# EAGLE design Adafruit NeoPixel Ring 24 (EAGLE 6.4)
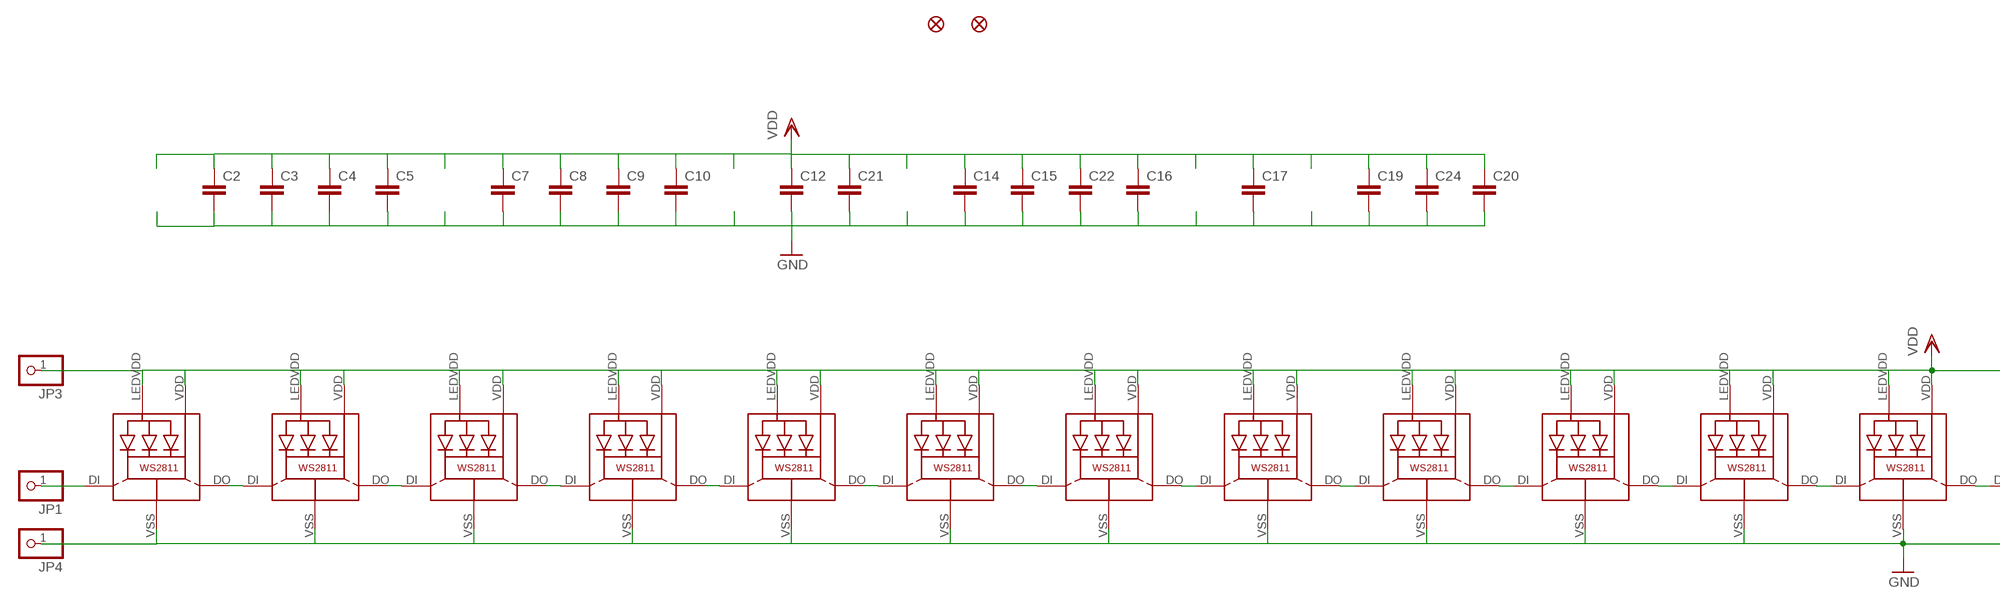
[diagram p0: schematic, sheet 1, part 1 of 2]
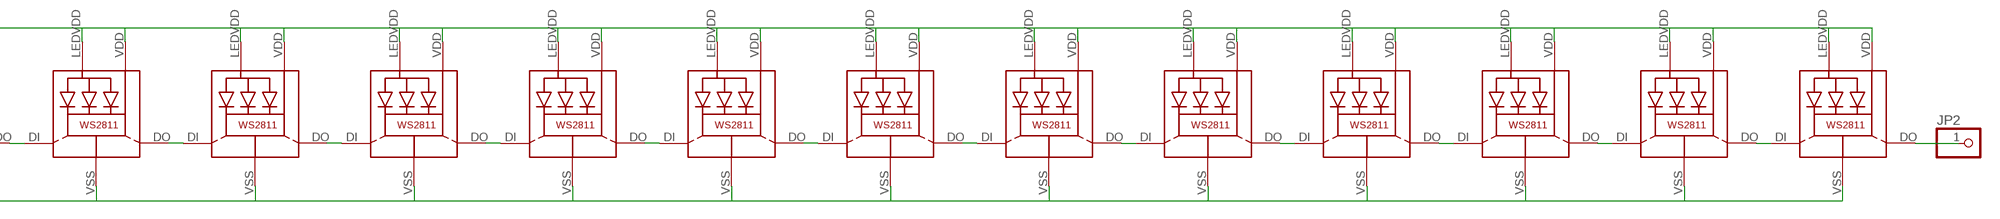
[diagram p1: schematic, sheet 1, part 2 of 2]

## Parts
C2  C-EUC0603  [C0603]
C3  C-EUC0603  [C0603]
C4  C-EUC0603  [C0603]
C5  C-EUC0603  [C0603]
C7  C-EUC0603  [C0603]
C8  C-EUC0603  [C0603]
C9  C-EUC0603  [C0603]
C10  C-EUC0603  [C0603]
C12  C-EUC0603  [C0603]
C14  C-EUC0603  [C0603]
C15  C-EUC0603  [C0603]
C16  C-EUC0603  [C0603]
C17  C-EUC0603  [C0603]
C19  C-EUC0603  [C0603]
C20  C-EUC0603  [C0603]
C21  C-EUC0603  [C0603]
C22  C-EUC0603  [C0603]
C24  C-EUC0603  [C0603]
FID1  FIDUCIAL""  [FIDUCIAL_1MM]
FID2  FIDUCIAL""  [FIDUCIAL_1MM]
JP1  PINHD-1X1CB  [1X01-CLEANBIG]
JP2  PINHD-1X1CB  [1X01-CLEANBIG]
JP3  PINHD-1X1CB  [1X01-CLEANBIG]
JP4  PINHD-1X1CB  [1X01-CLEANBIG]
LED1  WS28115050  [WS28115050]
LED2  WS28115050  [WS28115050]
LED3  WS28115050  [WS28115050]
LED4  WS28115050  [WS28115050]
LED5  WS28115050  [WS28115050]
LED6  WS28115050  [WS28115050]
LED7  WS28115050  [WS28115050]
LED8  WS28115050  [WS28115050]
LED9  WS28115050  [WS28115050]
LED10  WS28115050  [WS28115050]
LED11  WS28115050  [WS28115050]
LED12  WS28115050  [WS28115050]
LED13  WS28115050  [WS28115050]
LED14  WS28115050  [WS28115050]
LED15  WS28115050  [WS28115050]
LED16  WS28115050  [WS28115050]
LED17  WS28115050  [WS28115050]
LED18  WS28115050  [WS28115050]
LED19  WS28115050  [WS28115050]
LED20  WS28115050  [WS28115050]
LED21  WS28115050  [WS28115050]
LED22  WS28115050  [WS28115050]
LED23  WS28115050  [WS28115050]
LED24  WS28115050  [WS28115050]

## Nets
GND: C2.2 C3.2 C4.2 C5.2 C7.2 C8.2 C9.2 C10.2 C12.2 C14.2 C15.2 C16.2 C17.2 C19.2 C20.2 C21.2 C22.2 C24.2 JP4.1 LED1.VSS(GND) LED2.VSS(GND) LED3.VSS(GND) LED4.VSS(GND) LED5.VSS(GND) LED6.VSS(GND) LED7.VSS(GND) LED8.VSS(GND) LED9.VSS(GND) LED10.VSS(GND) LED11.VSS(GND) LED12.VSS(GND) LED13.VSS(GND) LED14.VSS(GND) LED15.VSS(GND) LED16.VSS(GND) LED17.VSS(GND) LED18.VSS(GND) LED19.VSS(GND) LED20.VSS(GND) LED21.VSS(GND) LED22.VSS(GND) LED23.VSS(GND) LED24.VSS(GND)
N$1: LED1.DO LED2.DI
N$2: LED2.DO LED3.DI
N$3: LED3.DO LED4.DI
N$4: LED4.DO LED5.DI
N$5: LED5.DO LED6.DI
N$6: LED6.DO LED7.DI
N$7: LED7.DO LED8.DI
N$8: LED8.DO LED9.DI
N$9: LED9.DO LED10.DI
N$10: LED10.DO LED11.DI
N$11: LED11.DO LED12.DI
N$12: LED12.DO LED13.DI
N$13: LED13.DO LED14.DI
N$14: LED14.DO LED15.DI
N$15: LED15.DO LED16.DI
N$16: LED16.DO LED17.DI
N$17: LED17.DO LED18.DI
N$18: LED18.DO LED19.DI
N$19: LED19.DO LED20.DI
N$20: LED20.DO LED21.DI
N$21: LED21.DO LED22.DI
N$22: LED22.DO LED23.DI
N$23: LED23.DO LED24.DI
N$24: JP2.1 LED24.DO
N$26: JP1.1 LED1.DI
VDD: C2.1 C3.1 C4.1 C5.1 C7.1 C8.1 C9.1 C10.1 C12.1 C14.1 C15.1 C16.1 C17.1 C19.1 C20.1 C21.1 C22.1 C24.1 JP3.1 LED1.LEDVDD LED1.VDD LED2.LEDVDD LED2.VDD LED3.LEDVDD LED3.VDD LED4.LEDVDD LED4.VDD LED5.LEDVDD LED5.VDD LED6.LEDVDD LED6.VDD LED7.LEDVDD LED7.VDD LED8.LEDVDD LED8.VDD LED9.LEDVDD LED9.VDD LED10.LEDVDD LED10.VDD LED11.LEDVDD LED11.VDD LED12.LEDVDD LED12.VDD LED13.LEDVDD LED13.VDD LED14.LEDVDD LED14.VDD LED15.LEDVDD LED15.VDD LED16.LEDVDD LED16.VDD LED17.LEDVDD LED17.VDD LED18.LEDVDD LED18.VDD LED19.LEDVDD LED19.VDD LED20.LEDVDD LED20.VDD LED21.LEDVDD LED21.VDD LED22.LEDVDD LED22.VDD LED23.LEDVDD LED23.VDD LED24.LEDVDD LED24.VDD

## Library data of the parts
C2-C5 C7-C10 C12 C14-C17 C19-C22 C24 = rcl:C-EU: CAPACITOR, European symbol
FID1 FID2 = microbuilder:FIDUCIAL: Fiducial Alignment Points; BOM: EXCLUDE
JP1-JP4 = NeoPixelRing:PINHD-1X1: Pin header 1x1 for 0.1" spacing
LED1-LED24 = microbuilder:WS28115050

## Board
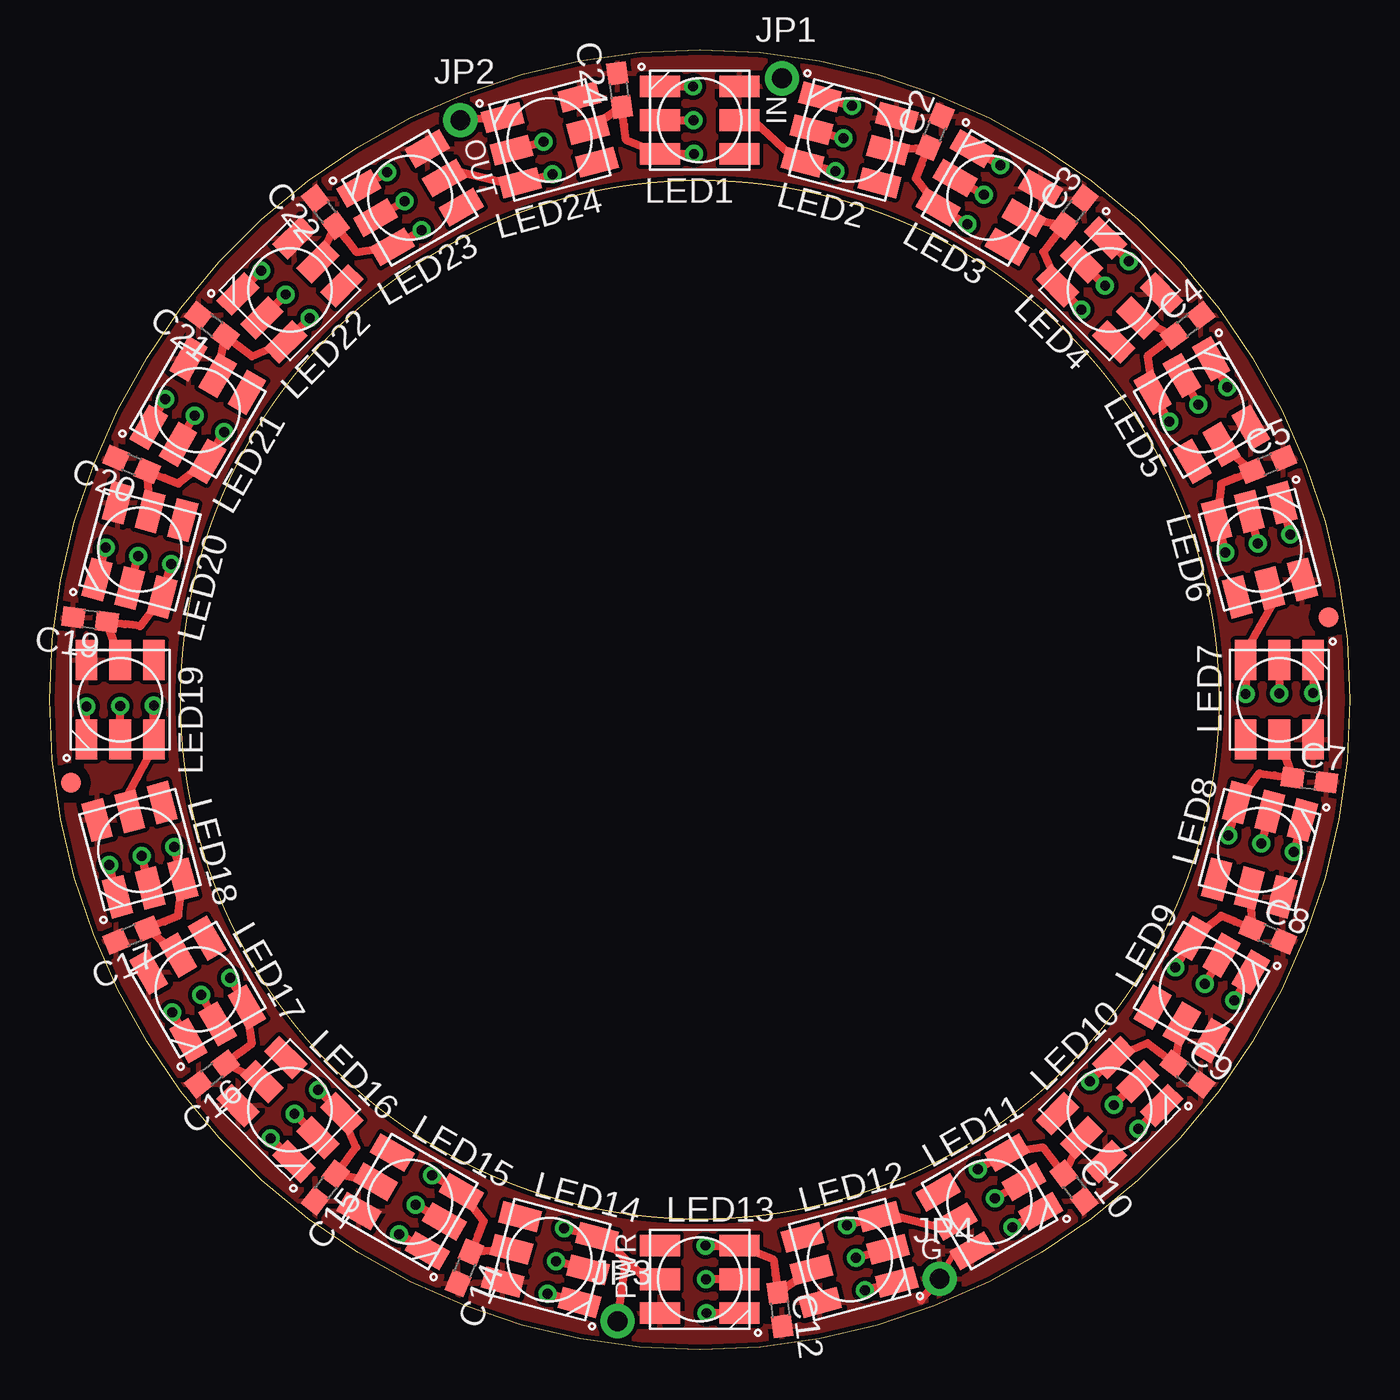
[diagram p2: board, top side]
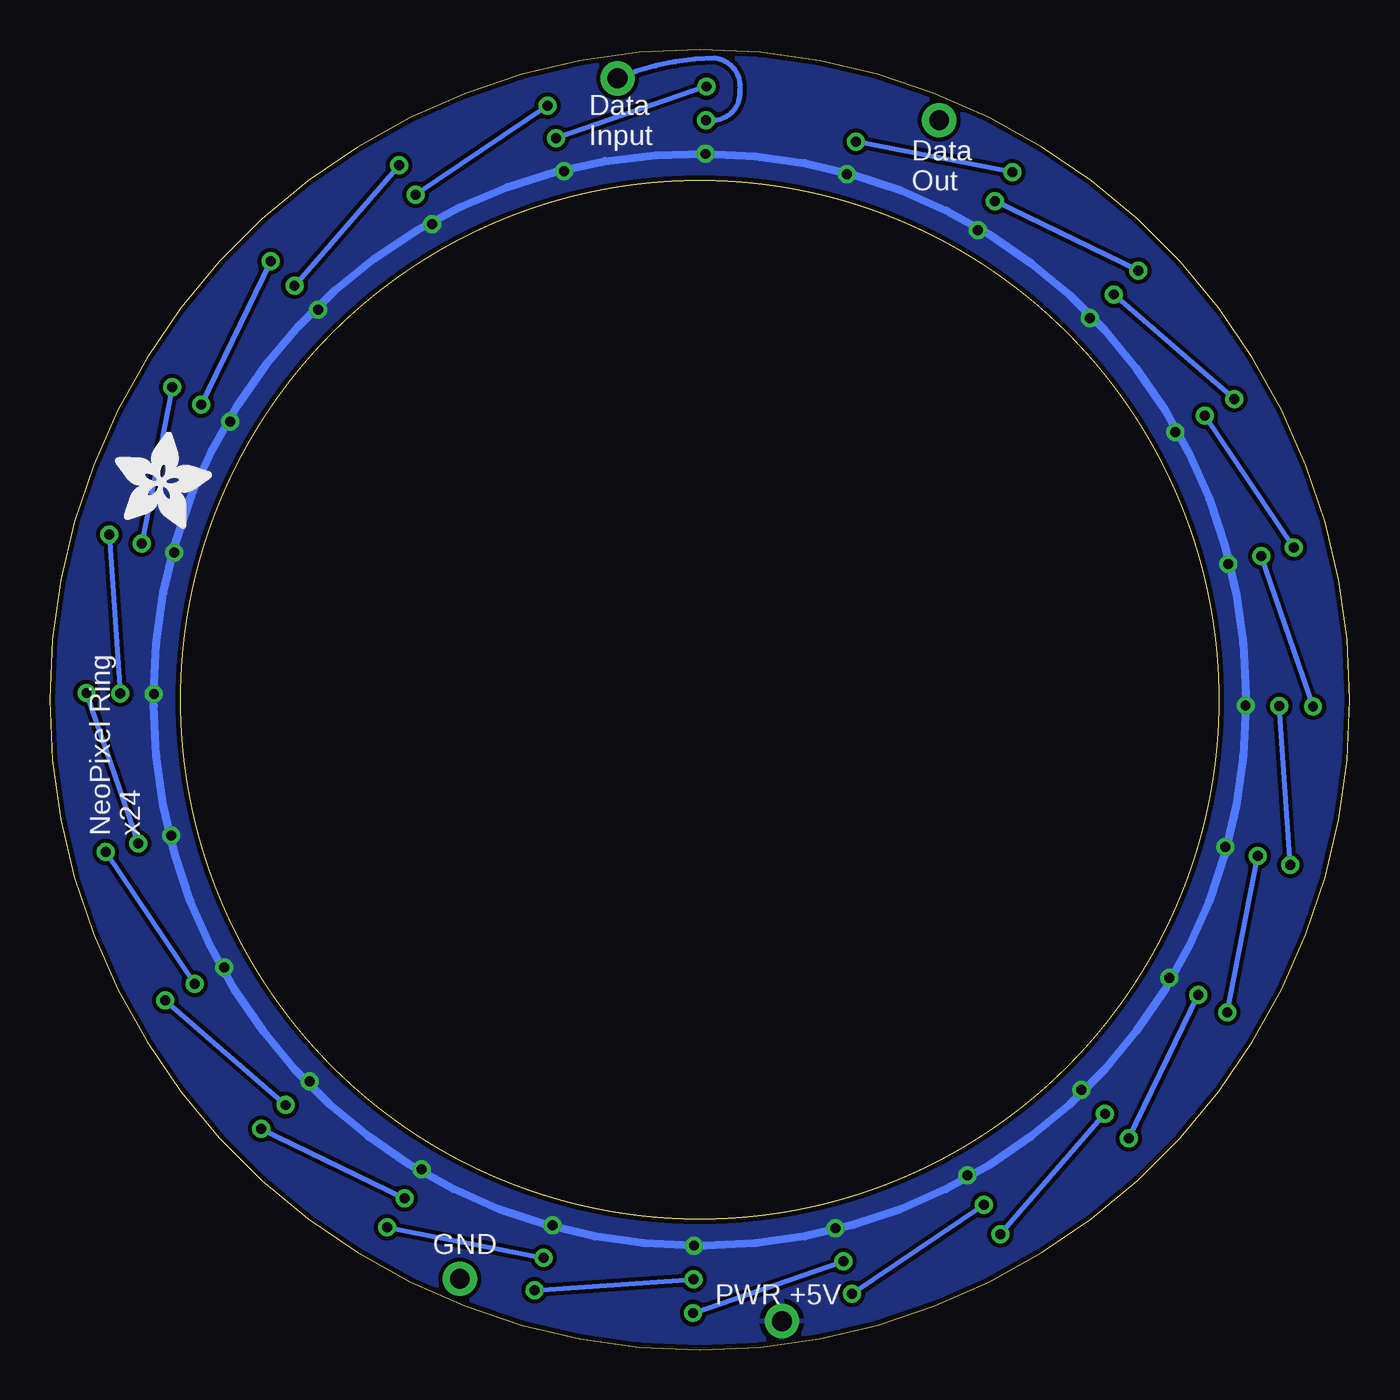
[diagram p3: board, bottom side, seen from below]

Size 65.53 x 65.53 mm. Coordinates in mm from the lower left corner, seen from the top.
Outline: 0,32.77 arc-90 32.77,65.53 arc-90 65.53,32.77 arc-90 32.77,0 arc-90 0,32.77
Outline: circle at 32.77,32.77 radius 26.16
Copper layers (1*16): Top 0.035mm / dielectric 1.5mm / Bottom 0.035mm
Design rules "adafruit": minimum track width 8mil, minimum drill 15.5mil, track to track 8mil, track to pad 8mil, pad to pad 8mil, via to via 8mil, smd to smd 8mil, copper to edge 10mil, drill to drill 8mil, minimum pad ring 10mil, minimum via ring 8mil, stop-mask expansion 4mil, vias tented up to drill 20mil, thermal gap 10mil
tRestrict: 1 lines

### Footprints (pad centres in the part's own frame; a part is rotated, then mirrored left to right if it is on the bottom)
C0603 = smd 1.1 x 1: 1 -0.85,0; 2 0.85,0
FIDUCIAL_1MM = smd 1 x 1: 1 0,0
1X01-CLEANBIG = drill 1 pad 1.727: 1 0,0
WS28115050 = smd 2 x 1.1: DI 2,0; DO 2,-1.7; LEDVDD -2,0; NC -2,1.7; VDD 2,1.7; VSS -2,-1.7

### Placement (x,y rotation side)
C2  44.62,61.4 67.5 top
C3  51.63,57.35 52.5 top
C4  57.35,51.63 37.5 top
C5  61.4,44.62 22.5 top
C7  63.49,28.72 352.5 top
C8  61.4,20.91 337.5 top
C9  57.35,13.9 322.5 top
C10  51.63,8.18 307.5 top
C12  36.81,2.04 277.5 top
C14  20.91,4.14 247.5 top
C15  13.9,8.18 232.5 top
C16  8.18,13.9 217.5 top
C17  4.14,20.91 202.5 top
C19  2.04,36.81 172.5 top
C20  4.14,44.62 157.5 top
C21  8.18,51.63 142.5 top
C22  13.9,57.35 127.5 top
C24  28.72,63.49 97.5 top
FID1  1.07,28.57 0 top
FID2  64.47,36.93 0 top
JP1  36.91,64.08 0 top
JP2  20.7,61.98 0 top
JP3  28.63,1.45 0 top
JP4  44.86,3.58 0 top
LED1  32.77,61.98 180 top
LED2  40.33,60.98 165 top
LED3  47.37,58.06 150 top
LED4  53.42,53.42 135 top
LED5  58.06,47.37 120 top
LED6  60.98,40.33 105 top
LED7  61.98,32.77 90 top
LED8  60.98,25.21 75 top
LED9  58.06,18.16 60 top
LED10  53.42,12.11 45 top
LED11  47.37,7.47 30 top
LED12  40.33,4.55 15 top
LED13  32.77,3.56 0 top
LED14  25.21,4.55 345 top
LED15  18.16,7.47 330 top
LED16  12.11,12.11 315 top
LED17  7.47,18.16 300 top
LED18  4.55,25.21 285 top
LED19  3.56,32.77 270 top
LED20  4.55,40.33 255 top
LED21  7.47,47.37 240 top
LED22  12.11,53.42 225 top
LED23  18.16,58.06 210 top
LED24  25.21,60.98 195 top
U$1  [ADAFRUIT_5MM]  62.23,41.4 0 bottom

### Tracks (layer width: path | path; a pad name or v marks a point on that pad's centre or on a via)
GND
  Top 0.305: JP4.1 45.59,4.93
  Top 0.406: 43.92,2.49 JP4.1
  pour Top: -18.03,83.57 -18.03,-18.03 83.57,-18.03 83.57,83.57
N$1  (via drill 0.5)
  Top 0.406: LED1.DO v32.43,63.67 | LED2.DI v40.02,61.06
  Bottom 0.254: v32.43,63.67 v40.02,61.06
N$2  (via drill 0.5)
  Top 0.406: LED2.DO v40.44,62.71 | LED3.DI v47.09,58.22
  Bottom 0.254: v40.44,62.71 v47.09,58.22
N$3  (via drill 0.5)
  Top 0.406: LED4.DI v53.19,53.64 | LED3.DO v47.93,59.7
  Bottom 0.254: v47.93,59.7 v53.19,53.64
N$4  (via drill 0.5)
  Top 0.406: LED5.DI v57.9,47.65 | LED4.DO v54.38,54.86
  Bottom 0.254: v54.38,54.86 v57.9,47.65
N$5  (via drill 0.5)
  Top 0.406: LED5.DO v59.36,48.51 | LED6.DI v60.9,40.63
  Bottom 0.254: v59.36,48.51 v60.9,40.63
N$6  (via drill 0.5)
  Top 0.406: LED6.DO v62.53,41.09 | LED7.DI v61.97,33.09
  Bottom 0.254: v62.53,41.09 v61.97,33.09
N$7  (via drill 0.5)
  Top 0.406: LED7.DO v63.67,33.1 | LED8.DI v61.06,25.51
  Bottom 0.254: v63.67,33.1 v61.06,25.51
N$8  (via drill 0.5)
  Top 0.406: LED8.DO v62.71,25.09 | LED9.DI v58.22,18.44
  Bottom 0.254: v62.71,25.09 v58.22,18.44
N$9  (via drill 0.5)
  Top 0.406: LED9.DO v59.7,17.6 | LED10.DI v53.64,12.34
  Bottom 0.254: v59.7,17.6 v53.64,12.34
N$10  (via drill 0.5)
  Top 0.406: LED10.DO v54.86,11.15 | LED11.DI v47.65,7.63
  Bottom 0.254: v54.86,11.15 v47.65,7.63
N$11  (via drill 0.5)
  Top 0.406: LED11.DO v48.51,6.17 | LED12.DI v40.63,4.63
  Bottom 0.254: v48.51,6.17 v40.63,4.63
N$12  (via drill 0.5)
  Top 0.406: LED12.DO v41.09,3 | LED13.DI v33.09,3.56
  Bottom 0.254: v41.09,3 v33.09,3.56
N$13  (via drill 0.5)
  Top 0.406: LED13.DO v33.1,1.86 | LED14.DI v25.51,4.47
  Bottom 0.254: v33.1,1.86 v25.51,4.47
N$14  (via drill 0.5)
  Top 0.406: LED14.DO v25.09,2.82 | LED15.DI v18.44,7.31
  Bottom 0.254: v25.09,2.82 v18.44,7.31
N$15  (via drill 0.5)
  Top 0.406: LED15.DO v17.6,5.83 | v12.34,11.89 LED16.DI
  Bottom 0.254: v17.6,5.83 v12.34,11.89
N$16  (via drill 0.5)
  Top 0.406: LED16.DO v11.15,10.67 | LED17.DI v7.63,17.89
  Bottom 0.254: v11.15,10.67 v7.63,17.89
N$17  (via drill 0.5)
  Top 0.406: LED17.DO v6.17,17.02 | LED18.DI v4.63,24.9
  Bottom 0.254: v6.17,17.02 v4.63,24.9
N$18  (via drill 0.5)
  Top 0.406: LED18.DO v3,24.44 | LED19.DI v3.56,32.45
  Bottom 0.254: v3,24.44 v3.56,32.45
N$19  (via drill 0.5)
  Top 0.406: LED19.DO v1.86,32.43 | LED20.DI v4.47,40.02
  Bottom 0.254: v1.86,32.43 v4.47,40.02
N$20  (via drill 0.5)
  Top 0.406: LED20.DO v2.82,40.44 | LED21.DI v7.31,47.09
  Bottom 0.254: v2.82,40.44 v7.31,47.09
N$21  (via drill 0.5)
  Top 0.406: LED21.DO v5.83,47.93 | LED22.DI v11.89,53.19
  Bottom 0.254: v5.83,47.93 v11.89,53.19
N$22  (via drill 0.5)
  Top 0.406: LED22.DO v10.67,54.38 | LED23.DI v17.89,57.9
  Bottom 0.254: v10.67,54.38 v17.89,57.9
N$23  (via drill 0.5)
  Top 0.406: LED23.DO v17.02,59.36 | LED24.DI v24.9,60.9
  Bottom 0.254: v17.02,59.36 v24.9,60.9
N$24
  Top 0.406: LED24.DO JP2.1
N$26  (via drill 0.5)
  Top 0.406: LED1.DI v32.45,61.97
  Bottom 0.254: v32.45,61.97 32.01,61.97 arc-90 30.73,63.5 arc-90 32,65.1 arc-22 JP1.1
VDD  (via drill 0.5)
  Top 0.406: LED24.LEDVDD C24.1 28.95,61.73 29.05,60.97 LED1.VDD v32.47,60.27 | v39.6,59.41 LED2.VDD 37.29,60.27 35.59,61.87 LED1.LEDVDD | v46.26,56.74 LED3.VDD 43.65,59.05 43.94,59.75 C2.1 LED2.LEDVDD | LED3.LEDVDD C3.1 50.55,55.94 50.08,55.33 LED4.VDD v52,52.43 | v56.44,46.78 LED5.VDD 55.33,50.08 55.94,50.55 C4.1 LED4.LEDVDD | LED5.LEDVDD C5.1 59.75,43.94 59.05,43.65 LED6.VDD v59.26,40.17 | LED7.LEDVDD C7.1 61.73,28.95 60.97,29.05 LED8.VDD v59.41,25.94 | LED8.LEDVDD C8.1 59.75,21.59 59.05,21.88 LED9.VDD v56.74,19.27 | LED9.LEDVDD C9.1 55.94,14.98 55.33,15.45 LED10.VDD v52.43,13.53 | LED10.LEDVDD C10.1 50.55,9.59 50.08,10.2 LED11.VDD v46.78,9.09 | v40.17,6.27 LED12.VDD 42.52,6.76 45.06,6.1 LED11.LEDVDD | LED12.LEDVDD C12.1 36.58,3.81 36.48,4.56 LED13.VDD v33.07,5.26 | v25.94,6.12 LED14.VDD 28.14,5.44 30.07,3.53 LED13.LEDVDD | LED14.LEDVDD C14.1 21.59,5.78 21.88,6.48 LED15.VDD v19.27,8.79 | LED15.LEDVDD C15.1 14.98,9.59 15.45,10.2 LED16.VDD v13.53,13.1 | LED16.LEDVDD C16.1 9.59,14.98 10.2,15.45 LED17.VDD v9.09,18.75 | LED17.LEDVDD C17.1 5.78,21.59 6.48,21.88 LED18.VDD v6.27,25.36 | LED19.LEDVDD C19.1 3.81,36.58 4.56,36.48 LED20.VDD v6.12,39.6 | LED20.LEDVDD C20.1 5.78,43.94 6.48,43.65 LED21.VDD v8.79,46.26 | v13.1,52 LED22.VDD 10.2,50.08 9.59,50.55 C21.1 LED21.LEDVDD | LED22.LEDVDD C22.1 14.98,55.94 15.45,55.33 LED23.VDD v18.75,56.44 | v25.36,59.26 LED24.VDD 23.04,58.8 20.68,59.38 LED23.LEDVDD | v5.26,32.47 LED19.VDD 5.03,29.95 3.94,27.96 LED18.LEDVDD | v60.27,33.07 LED7.VDD 60.5,35.61 61.67,37.64 LED6.LEDVDD | JP3.1 29.06,4.47
  Bottom 0.406: v32.47,60.27 arc90 5.26,33.07 v5.26,32.47 arc90 32.47,5.26 v33.07,5.26 arc90 60.27,32.47 v60.27,33.07 arc91 v32.47,60.27
  pour Bottom: -18.03,83.57 -18.03,-18.03 83.57,-18.03 83.57,83.57

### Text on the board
tPlace: IN | OUT | G | PWR
bPlace: Data / Input | Data / Out | NeoPixel Ring / x24 | GND | PWR +5V

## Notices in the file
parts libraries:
microbuilder: This work is placed in the public domain, and may be freely used for commercial and non-commercial work with the following conditions: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
